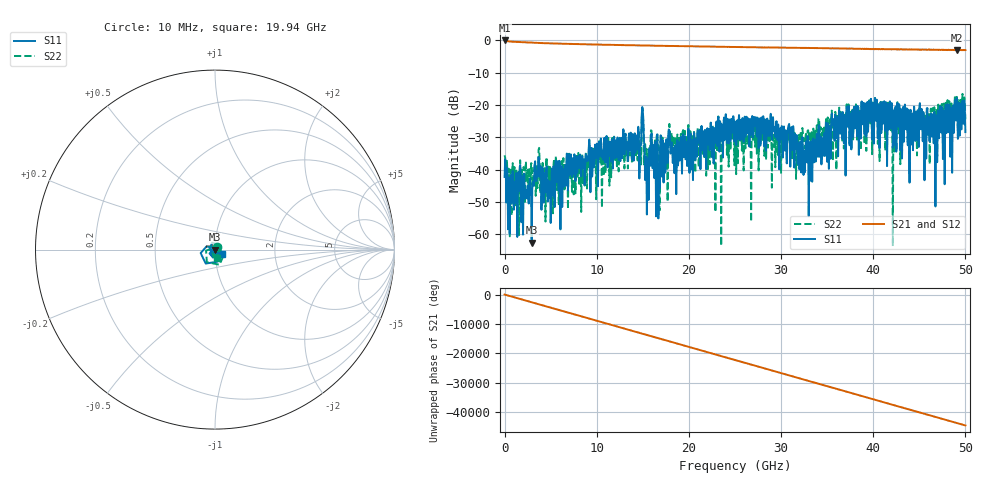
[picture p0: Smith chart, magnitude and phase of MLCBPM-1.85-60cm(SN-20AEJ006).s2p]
!Keysight Technologies,N5225A,MY51451228,A.10.40.14
!Date: Monday, March 22, 2021 13:50:18
!Correction: S11(Full 2 Port(1,3))
!S31(Full 2 Port(1,3))
!S13(Full 2 Port(1,3))
!S33(Full 2 Port(1,3))
!S2P File: Measurements: S11, S31, S13, S33:
# Hz S  dB  R 50
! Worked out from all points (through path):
!   801 points, 10 MHz to 50 GHz, reference 50 ohm
!   highest |S21| = -0.01 dB at 10 MHz (marker M1); lowest = -3.0 dB at 49.13 GHz (marker M2)
!   lowest |S11| = -62.7 dB at 2.947 GHz (marker M3), VSWR 1.00, Z = 49.9 - j0.0214 ohm
!   |S11| at or under -10 dB: start of sweep to end of sweep
!   |S22| runs from -63.7 to -16.5 dB; largest |S21 - S12| = 0.0051
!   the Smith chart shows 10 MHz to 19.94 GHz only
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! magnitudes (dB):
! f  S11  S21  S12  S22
! 10 MHz  -42.2  0.0  0.0  -35.6
! 572.4 MHz  -59.9  -0.3  -0.3  -60.7
! 2.947 GHz  -62.7  -0.7  -0.7  -38.1
! 3.509 GHz  -40.6  -0.8  -0.7  -38.9
! 4.884 GHz  -47.7  -0.9  -0.9  -47.3
! 8.383 GHz  -36.4  -1.2  -1.2  -36.8
! 14.94 GHz  -20.6  -1.6  -1.6  -21.1
! 15.38 GHz  -35.9  -1.6  -1.6  -35.4
! 15.94 GHz  -28.9  -1.6  -1.6  -27.9
! 16.69 GHz  -55.1  -1.6  -1.6  -33.5
! 17.82 GHz  -27.6  -1.7  -1.7  -28.2
! 18.63 GHz  -47.6  -1.7  -1.7  -41.1
! 25 GHz  -25.1  -2.0  -2.0  -25.8
! 29.07 GHz  -25.3  -2.2  -2.2  -26.4
! 33.38 GHz  -43.7  -2.3  -2.3  -31.0
! 35.69 GHz  -24.4  -2.5  -2.4  -25.6
! 41.69 GHz  -27.6  -2.7  -2.7  -27.8
! 42.31 GHz  -32.4  -2.7  -2.7  -34.4
! 42.63 GHz  -19.4  -2.8  -2.8  -19.1
! 46.75 GHz  -51.4  -2.9  -2.8  -36.1
! 49.13 GHz  -19.9  -3.0  -3.0  -19.7
! 50 GHz  -28.4  -3.0  -3.0  -24.4
